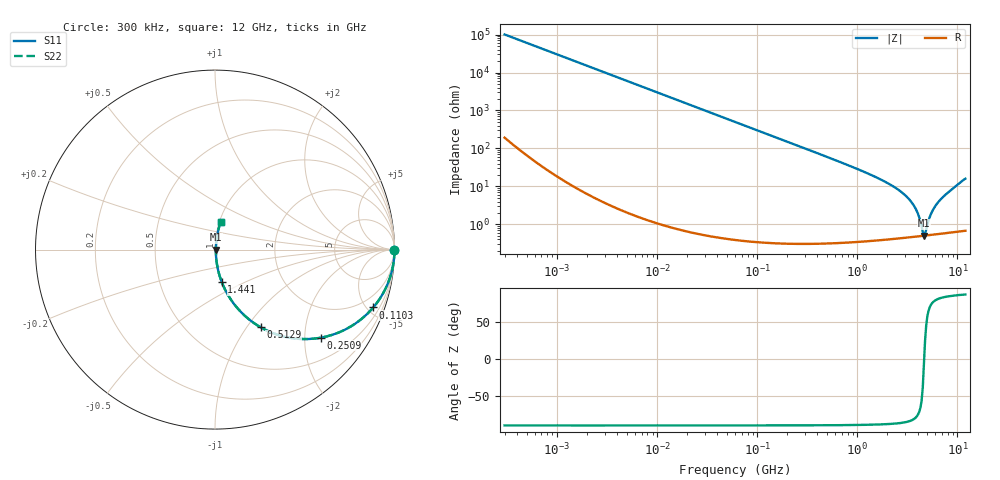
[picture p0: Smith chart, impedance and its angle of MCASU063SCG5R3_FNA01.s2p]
! MCASU063SCG5R3_FNA01  S-PARAMETER MODEL  ( General Type )
! Model Generated by TAIYO YUDEN Corporation (http://www.ty-top.com)
! Version 1.0
! TAIYO YUDEN Control No. 130801
! Copyright(c) 2013 TAIYO YUDEN CO.,LTD. All Rights Reserved.
! Product Description (link to TY-COMPAS)
! https://ds.yuden.co.jp/TYCOMPAS/or/detail?pn=MCASU063SCG5R3DFNA01&u=M
! Products Name : Multilayer Ceramic Capacitors
! Characteristics :
!  Capacitance : 5.3 pF , Rated Voltage : 50V , TCC : CG / C0G
!  Case Size : 0.6 x 0.3 / 0.024 x 0.012 [mm/inch] , Thickness : 0.3 / 0.012 [mm/inch]
!  (Conditions: Temperature = 25 degC , DC Bias Current/Voltage = 0A / 0V)
! External Node Assignments :
!  1  o---| |---o  2
! GND o---------o GND
! Frequency Range : 0.3MHz  -  12000MHz  [ 401 STEP ]
# MHz S RI R 50
! Freq[MHz].  S11 Real  S11 Imag  S21 Real  S21 Imag  S12 Real  S12 Imag  S22 Real  S22 Imag
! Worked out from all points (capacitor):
!   401 points, 300 kHz to 12 GHz, reference 50 ohm
!   read as one part in series: C = 5.28 pF near 316.3 kHz
!   lowest |Z| = 504 mohm at 4.624 GHz (marker M1)
!   series resonance near 4.643 GHz, so ESL is about 220 pH
!   S11 on the Smith chart (normalised r, x): 300 kHz: open; 110.3 MHz: 1.01, -5.46; 250.9 MHz: 1.01, -2.40; 512.9 MHz: 1.01, -1.16; 1.441 GHz: 1.01, -0.38; 12 GHz: 1.01, +0.32
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0.3  1 -0.000994  2.89e-06 0.000994  2.89e-06 0.000994  1 -0.000994
1.769972  1 -0.00587  3.7e-05 0.00587  3.7e-05 0.00587  1 -0.00587
10.44266  0.9988 -0.0346  0.00121 0.0346  0.00121 0.0346  0.9988 -0.0346
27.82928  0.9915 -0.0915  0.00848 0.0915  0.00848 0.0915  0.9915 -0.0915
60  0.9618 -0.1913  0.0382 0.1913  0.0382 0.1913  0.9618 -0.1913
110.3493  0.8816 -0.3225  0.1184 0.3225  0.1184 0.3225  0.8816 -0.3225
250.8588  0.5896 -0.4906  0.4104 0.4906  0.4104 0.4906  0.5896 -0.4906
353.9943  0.4182 -0.4915  0.5818 0.4915  0.5818 0.4915  0.4182 -0.4915
512.9422  0.2535 -0.4323  0.7465 0.4323  0.7465 0.4323  0.2535 -0.4323
826.3444  0.1134 -0.3124  0.8866 0.3124  0.8866 0.3124  0.1134 -0.3124
1441.349  0.0378 -0.1813  0.9622 0.1813  0.9622 0.1813  0.0378 -0.1813
2088.533  0.017 -0.1128  0.983 0.1128  0.983 0.1128  0.017 -0.1128
2795.104  0.00898 -0.0679  0.991 0.0679  0.991 0.0679  0.00898 -0.0679
3454.93  0.00609 -0.0385  0.9939 0.0385  0.9939 0.0385  0.00609 -0.0385
3944.255  0.00522 -0.0211  0.9948 0.0211  0.9948 0.0211  0.00522 -0.0211
4502.883  0.00497 -0.00394  0.995 0.00394  0.995 0.00394  0.00497 -0.00394
4623.766  0.005 -0.000444  0.995 0.000444  0.995 0.000444  0.005 -0.000444
4875.354  0.00511 0.00527  0.9949 -0.00527  0.9949 -0.00527  0.00511 0.00527
5565.855  0.00571 0.0205  0.9943 -0.0205  0.9943 -0.0205  0.00571 0.0205
6354.153  0.00684 0.0363  0.9932 -0.0363  0.9932 -0.0363  0.00684 0.0363
7854.144  0.01 0.0639  0.99 -0.0639  0.99 -0.0639  0.01 0.0639
12000  0.0309 0.153  0.9691 -0.153  0.9691 -0.153  0.0309 0.153
